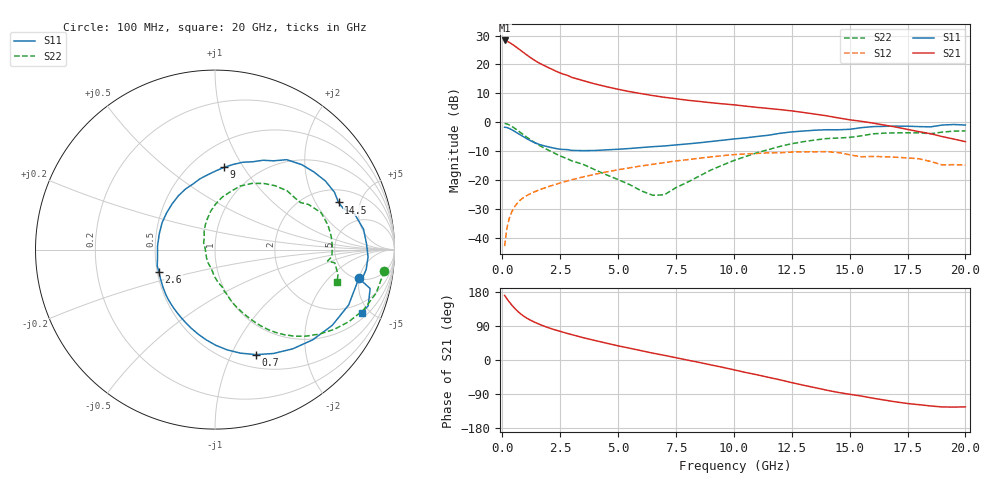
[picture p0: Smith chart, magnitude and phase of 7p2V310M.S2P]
! Infineon Technologies  Discrete & RF Semiconductors
! bfp620
! VCE =  2.3 V,  IC =  10 mA
! Common Emitter S-Parameters:  Sep 2002
# GHz  S  MA  R  50
!  f  S11  S21  S12  S22
! GHz  MAG  ANG  MAG  ANG  MAG  ANG  MAG  ANG
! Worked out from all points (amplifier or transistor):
!   59 points, 100 MHz to 20 GHz, reference 50 ohm
!   highest |S21| = 28.3 dB at 100 MHz (marker M1)
!   |S21| within 3 dB of that: start of sweep to 720.3 MHz
!   unconditionally stable (mu >= 1): 3.941 GHz to 10.84 GHz; 17.14 GHz to end of sweep
!   at 1 GHz: K = 0.51, MSG = 24.7 dB, |S12| = -25.7 dB
!   at 5.5 GHz: K = 1.05, MAG = 11.8 dB, |S12| = -15.8 dB
!   at 20 GHz: K = 1.29, MAG = 0.8 dB, |S12| = -14.9 dB
!   S11 on the Smith chart (normalised r, x): 100 MHz: 5.24, -4.94; 700 MHz: 0.65, -1.25; 2.6 GHz: 0.51, -0.14; 9 GHz: 0.71, +0.83; 14.5 GHz: 2.75, +3.16; 20 GHz: 1.31, -4.46
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0.1  0.818 -11.0  25.98 170.6  0.0071 64.0  0.9506 -7.2
0.2  0.8061 -22.5  25.21 161.5  0.0146 70.7  0.93 -15.1
0.3  0.7776 -32.9  24.06 153.3  0.0214 68.9  0.8935 -22.0
0.4  0.7411 -42.7  22.73 145.7  0.0274 66.0  0.8481 -28.2
0.5  0.7024 -51.9  21.34 138.8  0.0327 63.0  0.7989 -33.8
0.6  0.6644 -60.6  19.97 132.4  0.0375 60.2  0.749 -38.9
0.7  0.6284 -68.6  18.66 126.6  0.0416 57.8  0.7004 -43.5
0.8  0.5945 -76.1  17.41 121.4  0.0454 55.7  0.6542 -47.5
1  0.5332 -89.5  15.16 112.6  0.0518 52.4  0.5705 -53.9
1.2  0.4814 -101.0  13.26 105.6  0.0573 50.0  0.5 -58.7
1.4  0.4406 -111.3  11.73 99.7  0.0623 48.3  0.4423 -62.4
1.9  0.3803 -133.3  9.168 87.2  0.0742 45.3  0.341 -69.5
2.6  0.3366 -158.6  6.854 73.8  0.0908 41.7  0.25 -75.9
3.5  0.3207 175.9  5.223 58.8  0.1128 36.4  0.185 -84.3
5  0.3388 142.5  3.707 37.4  0.1496 25.7  0.1013 -104.1
7  0.386 108.3  2.693 12.3  0.1991 9.7  0.0552 173.6
9  0.4612 83.6  2.173 -12.8  0.2495 -9.4  0.1473 111.6
10.5  0.5333 66.6  1.894 -32.8  0.2809 -26.6  0.2534 89.3
13.5  0.7245 31.8  1.377 -72.9  0.3061 -60.2  0.4899 46.5
14.5  0.7367 20.9  1.185 -85.5  0.2976 -75.0  0.5297 33.1
17  0.8536 -2.7  0.821 -110.6  0.2461 -91.5  0.6517 6.5
20  0.8902 -23.4  0.459 -123.8  0.1802 -102.8  0.7045 -14.8
